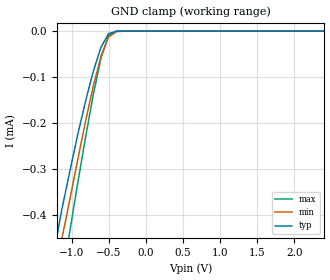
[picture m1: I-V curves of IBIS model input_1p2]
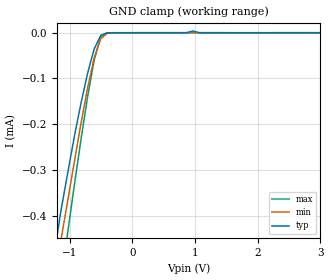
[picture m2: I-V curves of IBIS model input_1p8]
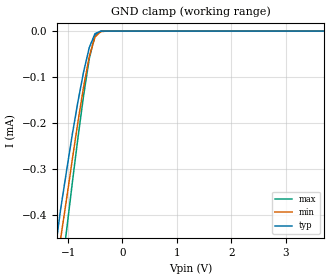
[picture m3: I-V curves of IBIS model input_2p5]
| Texas Instruments Incorporated
| TXU0102 Single-Bit Fixed Direction Voltage-Level Translator
| with 3-State outputs and Schmitt-trigger Inputs
[IBIS Ver]   4.1
[File name]   txu0102.ibs
[File Rev]   1.0
[Date]   11/16/2021
[Source]
| Texas Instruments Incorporated.
| Analog-eLab Design Center, HPA
| 12500 TI Blvd
| Dallas, TX -75243
[Notes]   Revision History:
[Disclaimer]
| This model is designed as an aid for customers of Texas Instruments.
| TI and its licensors and suppliers make no warranties, either expressed
| or implied, with respect to this  model, including the warranties of
| merchantability or fitness for a particular purpose. The model is
| provided solely on an "as is" basis. The entire risk as to its quality
| and performance is with the customer.
| This model is subject to change without notice. Texas Instruments
| Incorporated is not responsible for updating this model.
[Copyright]
 (C) Copyright 2021 Texas Instruments Incorporated.All rights reserved.
|  Component TXU0102DCU 8-Pin VSSOP - DCU package
|  Part # TXU0102DCU
[Component]   TXU0102DCU
[Manufacturer]   TI
[Package]   |8 VSSOP - DCU package
|   typ   min   max
R_pkg   3.900e-02   3.000e-02   4.600e-02
L_pkg   2.685e-09   2.367e-09   3.177e-09
C_pkg   3.200e-13   2.520e-13   4.340e-13
[Pin]   signal_name   model_name   R_pin   L_pin   C_pin
1   B2Y   output   4.600e-02   2.532e-09   2.570e-13
2   GND   gnd   3.700e-02   2.670e-09   3.460e-13
3   VCCA   power   3.700e-02   3.153e-09   4.340e-13
4   A2   input   4.200e-02   2.741e-09   2.900e-13
5   A1   input   4.200e-02   2.741e-09   2.900e-13
6   OE   input   3.100e-02   2.738e-09   3.390e-13
7   VCCB   power   3.600e-02   2.653e-09   3.440e-13
8   B1Y   output   4.200e-02   2.648e-09   2.820e-13
|  Component TXU0102SON 8-Pin SON - DTT package
|  Part # TXU0102DTT
[Component]   TXU0102DTT
[Manufacturer]   TI
[Package]   |8 SON - DTT package
|   typ   min   max
R_pkg   3.700e-02   2.500e-02   5.300e-02
L_pkg   8.060e-10   5.310e-10   1.139e-09
C_pkg   1.880e-13   5.700e-14   3.100e-13
[Pin]   signal_name   model_name   R_pin   L_pin   C_pin
1   B2Y   output   4.600e-02   2.532e-09   2.570e-13
2   GND   gnd   3.700e-02   2.670e-09   3.460e-13
3   VCCA   power   3.700e-02   3.153e-09   4.340e-13
4   A2   input   4.200e-02   2.741e-09   2.900e-13
5   A1   input   4.200e-02   2.741e-09   2.900e-13
6   OE   input   3.100e-02   2.738e-09   3.390e-13
7   VCCB   power   3.600e-02   2.653e-09   3.440e-13
8   B1Y   output   4.200e-02   2.648e-09   2.820e-13
|  Component TXU0102SON 8-Pin X2SON - DTM package
|  Part # TXU0102DTM
[Component]   TXU0102DTM
[Manufacturer]   TI
[Package]   |8 X2SON - DTM package
|   typ   min   max
R_pkg   3.700e-02   2.500e-02   5.300e-02
L_pkg   8.060e-10   5.310e-10   1.139e-09
C_pkg   1.880e-13   5.700e-14   3.100e-13
[Pin]   signal_name   model_name   R_pin   L_pin   C_pin
1   B2Y   output   4.600e-02   2.532e-09   2.570e-13
2   GND   gnd   3.700e-02   2.670e-09   3.460e-13
3   VCCA   power   3.700e-02   3.153e-09   4.340e-13
4   A2   input   4.200e-02   2.741e-09   2.900e-13
5   A1   input   4.200e-02   2.741e-09   2.900e-13
6   OE   input   3.100e-02   2.738e-09   3.390e-13
7   VCCB   power   3.600e-02   2.653e-09   3.440e-13
8   B1Y   output   4.200e-02   2.648e-09   2.820e-13
|   Model Selectors
[Model Selector] input
input_1p2   1.2V   digital input
input_1p8   1.8V   digital input
input_2p5   2.5V   digital input
input_3p3   3.3V   digital input
input_5p0   5.0V   digital input
[Model Selector] output
output_1p2   1.2V   digital output
output_1p8   1.8V   digital output
output_2p5   2.5V   digital output
output_3p3   3.3V   digital output
output_5p0   5.0V   digital output
| Models and submodels in the file (10): input_1p2 (Input), input_1p8 (Input), input_2p5 (Input), input_3p3 (Input), input_5p0 (Input), output_1p2 (Output), output_1p8 (Output), output_2p5 (Output), output_3p3 (Output), output_5p0 (Output)
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|   input_1p2 Model
[Model]   input_1p2
Model_type   Input
Vinl = 0.2
Vinh = 0.9
|   typ   min   max
C_comp   0.119pF   0.105pF   0.126pF
[Voltage Range]   1.2   1.08   1.32
|Junction Temperature
[Temperature Range]   25   125   -40
[GND Clamp Reference]   0   0   0
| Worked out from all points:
|   GND clamp passes 1 mA (typ) near -1.81 V on its own axis
[GND Clamp]
|   Voltage   I(typ)   I(min)   I(max)
-2.5V     -1.66mA    -1.64mA    -2.09mA
-1.24V    -478uA     -541uA     -650uA
-1.14V    -389uA     -453uA     -542uA
-1.03V    -305uA     -366uA     -435uA
-925mV    -226uA     -281uA     -332uA
-820mV    -154uA     -198uA     -233uA
-715mV    -88.7uA    -121uA     -140uA
-610mV    -35.6uA    -54.9uA    -59.7uA
-505mV    -5.5uA     -12.7uA    -8.49uA
-400mV    -210nA     -1.13uA    -141nA
8V        3.62nA     3.43nA     4.23nA
|   input_1p8 Model
[Model]   input_1p8
Model_type   Input
Vinl = 0.7
Vinh = 1.1
|   typ   min   max
C_comp   3.13pF   2.65pF   3.82pF
| Where Nom  PVT is Nominal Process, 2.25V, 27C
|   Fast PVT is Strong Process,  2.50V, -55C
|   Slow PVT is Weak Process,   2.0V, 150C
[Voltage Range]   1.8   1.62   1.98
|Junction Temperature
[Temperature Range]   25   125   -40
[GND Clamp Reference]   0   0   0
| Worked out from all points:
|   GND clamp passes 1 mA (typ) near -1.81 V on its own axis
[GND Clamp]
|   Voltage   I(typ)   I(min)   I(max)
-2.5V     -1.66mA    -1.64mA    -2.09mA
-1.24V    -478uA     -541uA     -650uA
-1.14V    -389uA     -453uA     -542uA
-1.03V    -305uA     -366uA     -435uA
-820mV    -154uA     -198uA     -233uA
-715mV    -88.7uA    -121uA     -140uA
-610mV    -35.6uA    -54.9uA    -59.7uA
-505mV    -5.5uA     -12.7uA    -8.49uA
-400mV    -210nA     -1.13uA    -141nA
965mV     3.74uA     3.02nA     4.93nA
1.07V     3.25nA     2.95nA     3.92nA
8V        3.62nA     3.43nA     4.23nA
|   input_2p5 Model
[Model]   input_2p5
Model_type   Input
Vinl = 1.0
Vinh = 1.4
|   typ   min   max
C_comp   3.03pF   2.54pF   3.83pF
| Where Nom  PVT is Nominal Process, 2.25V, 27C
|   Fast PVT is Strong Process,  2.50V, -55C
|   Slow PVT is Weak Process,   2.0V, 150C
[Voltage Range]   2.5   2.25   2.75
|Junction Temperature
[Temperature Range]   25   125   -40
[GND Clamp Reference]   0   0   0
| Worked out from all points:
|   GND clamp passes 1 mA (typ) near -1.81 V on its own axis
[GND Clamp]
|   Voltage   I(typ)   I(min)   I(max)
-2.5V     -1.66mA    -1.64mA    -2.09mA
-1.24V    -478uA     -541uA     -650uA
-1.14V    -389uA     -453uA     -542uA
-1.03V    -305uA     -366uA     -435uA
-925mV    -226uA     -281uA     -332uA
-820mV    -154uA     -198uA     -233uA
-715mV    -88.7uA    -121uA     -140uA
-610mV    -35.6uA    -54.9uA    -59.7uA
-505mV    -5.5uA     -12.7uA    -8.49uA
-400mV    -210nA     -1.14uA    -141nA
8V        3.62nA     3.43nA     4.23nA
